ORGANIZATION_BLOCK MAIN:OB1
TITLE= Inversione di Marcia con Temporizzatore di Blocco
// Simulatore: 01
// VERSIONE: 1.0
// DATA: 26/02/2002
//
// Questo esempio di programmazione spiega come controllare un motore
// trifase caratterizzato da due sensi di rotazione.
// Il pulsante SB3 consente di avviare il motore in
// senso antiorario, il pulsante nell'ingresso SB2 consente di
// avviarlo in senso orario.
// Per poter procedere è necessario che il salvamotore FR  e il
// pulsante di STOP (SB1) siano disattivati.
// Il senso di rotazione può essere invertito solo dopo che è stato
// premuto il pulsante STOP (SB1) e  sono trascorsi 5 s.
// Ciò consente al motore di frenare e riavviarsi nella direzione
// opposta.
//

BEGIN
NETWORK 1 // Imposta l'interblocco
LD M1.0
S M2.0 1

NETWORK 2 // Resetta l'interblocco
LDN M1.0
R M2.0 1

NETWORK 3 // Aziona in senso antiorario
LD I0.3
O I0.4
AN M2.0
AN I0.0
A I0.1
A I0.5
= Q0.1
= Q0.4

NETWORK 4 // Aziona in senso orario
LD I0.2
O I0.0
AN M2.0
AN I0.4
A I0.1
A I0.5
= Q0.0
= Q0.3

NETWORK 5 // Segnalazione Motore Fermo
LDN Q0.0
AN Q0.1
= Q0.2

NETWORK 6 // Imposta il bit di temporizzazione del tempo di attesa
LD Q0.0
O Q0.1
ED
S M1.0 1

NETWORK 7 // Imposta il temporizzatore del tempo di attesa
LD M1.0
TON T33 +50
A T33
R M1.0 1

NETWORK 8 //Lampeggio lampada  spia durante il tempo di attesa
//
LD M1.0
A SM0.5
= Q0.6

NETWORK 9 //Segnalazione Relè Termico Scattato
//
LDN I0.5
= Q0.5

END_ORGANIZATION_BLOCK

